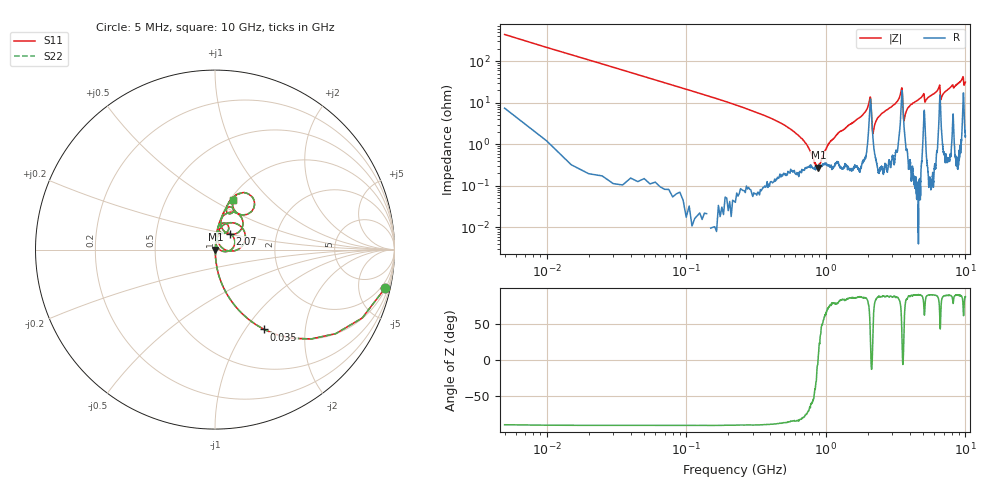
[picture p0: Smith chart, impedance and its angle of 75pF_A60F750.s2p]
! Amotech Co.,Ltd.
! http://www.amotech.co.kr/
! Part Number: A60F750
! These Parameters are Measured in Series Mode Connection
! Operation Temp=25[degC], DC Bias Voltage=0[V]
! Freq. Start=5[MHz] Stop=10[GHz], 2000[Steps]
! Date: Monday, July 20, 2020, 03:43:29
# GHZ S RI R 50.000000
!Freq.(Hz) S11(Real) S11(Imag) S21(Real) S21(Imag) S12(Real) S12(Imag) S22(Real) S22(Imag)
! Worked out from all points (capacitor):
!   2000 points, 5 MHz to 10 GHz, reference 50 ohm
!   read as one part in series: C = 74.1 pF near 55 MHz
!   lowest |Z| = 272 mohm at 885 MHz (marker M1)
!   series resonance near 880.6 MHz, so ESL is about 440 pH
!   S11 on the Smith chart (normalised r, x): 5 MHz: 1.15, -8.80; 35 MHz: 1.00, -1.23; 2.07 GHz: 1.16, +0.21; 10 GHz: 1.03, +0.63
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0.005  0.9476 -0.2145  0.0524 0.2145  0.0524 0.2145  0.9476 -0.2145
0.035  0.2737 -0.445  0.7263 0.445  0.7263 0.445  0.2737 -0.445
0.075  0.0754 -0.2627  0.9246 0.2627  0.9246 0.2627  0.0754 -0.2627
0.135  0.0238 -0.1517  0.9762 0.1517  0.9762 0.1517  0.0238 -0.1517
0.67  0.00227 -0.0138  0.9977 0.0138  0.9977 0.0138  0.00227 -0.0138
0.885  0.0027 0.000339  0.9973 -0.000339  0.9973 -0.000339  0.0027 0.000339
1.2  0.00387 0.0167  0.9961 -0.0167  0.9961 -0.0167  0.00387 0.0167
1.675  0.00457 0.0399  0.9954 -0.0399  0.9954 -0.0399  0.00457 0.0399
2.07  0.0832 0.088  0.9168 -0.088  0.9168 -0.088  0.0832 0.088
2.195  0.0106 0.0178  0.9894 -0.0178  0.9894 -0.0178  0.0106 0.0178
2.43  0.00451 0.0482  0.9955 -0.0482  0.9955 -0.0482  0.00451 0.0482
3.34  0.0292 0.1184  0.9708 -0.1184  0.9708 -0.1184  0.0292 0.1184
3.5  0.1581 0.1117  0.8419 -0.1117  0.8419 -0.1117  0.1581 0.1117
3.645  0.0241 0.0291  0.9759 -0.0291  0.9759 -0.0291  0.0241 0.0291
3.905  0.00914 0.0766  0.9909 -0.0766  0.9909 -0.0766  0.00914 0.0766
5.005  0.0479 0.1487  0.9521 -0.1487  0.9521 -0.1487  0.0479 0.1487
5.155  0.0292 0.098  0.9708 -0.098  0.9708 -0.098  0.0292 0.098
6.51  0.1165 0.205  0.8835 -0.205  0.8835 -0.205  0.1165 0.205
6.67  0.0569 0.0976  0.9431 -0.0976  0.9431 -0.0976  0.0569 0.0976
8.335  0.0643 0.2254  0.9357 -0.2254  0.9357 -0.2254  0.0643 0.2254
9.65  0.2196 0.2649  0.7804 -0.2649  0.7804 -0.2649  0.2196 0.2649
10  0.1012 0.2771  0.8988 -0.2771  0.8988 -0.2771  0.1012 0.2771
